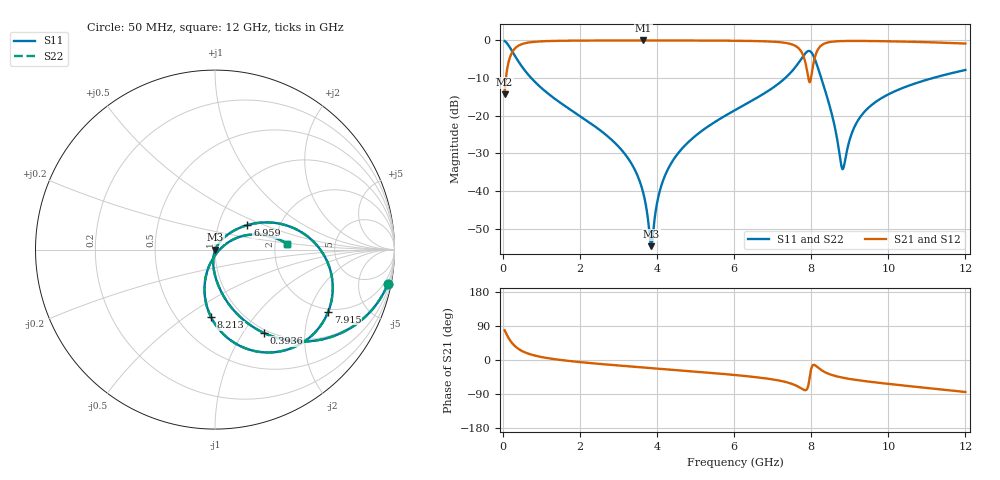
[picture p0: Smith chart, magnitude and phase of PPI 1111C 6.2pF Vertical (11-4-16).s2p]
# GHz S MA R 50
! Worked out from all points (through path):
!   1601 points, 50 MHz to 12 GHz, reference 50 ohm
!   highest |S21| = -0.02 dB at 3.65 GHz (marker M1); lowest = -14.3 dB at 50 MHz (marker M2)
!   group delay of S21, straight-line fit = 22.8 ps
!   lowest |S11| = -54.6 dB at 3.852 GHz (marker M3), VSWR 1.00, Z = 50.2 - j0.0771 ohm
!   |S11| at or under -10 dB: 741.6 MHz to 7.326 GHz (6.585 GHz wide, 163 % of centre); 8.262 GHz to 11.15 GHz (2.891 GHz wide, 29.8 % of centre)
!   |S22| runs from -54.6 to -0.2 dB; largest |S21 - S12| = 0
!   S11 on the Smith chart (normalised r, x): 50 MHz: 0.95, -9.92; 393.6 MHz: 0.95, -1.25; 6.959 GHz: 1.37, +0.40; 7.915 GHz: 1.89, -2.70; 8.213 GHz: 0.72, -0.64; 12 GHz: 2.34, +0.18
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0.05  0.9812 -11.4  0.1929 78.6  0.1929 78.6  0.9812 -11.4
0.1919063  0.7976 -38.2  0.6029 51.8  0.6029 51.8  0.7976 -38.2
0.3935625  0.5396 -59.5  0.8414 30.4  0.8414 30.4  0.5396 -59.5
0.8715625  0.2701 -79.0  0.9619 10.8  0.9619 10.8  0.2701 -79.0
2.044156  0.09594 -95.2  0.994 -5.9  0.994 -5.9  0.09594 -95.2
3.142063  0.03237 -102.8  0.9977 -15.6  0.9977 -15.6  0.03237 -102.8
3.649938  0.009261 -98.6  0.998 -19.7  0.998 -19.7  0.009261 -98.6
3.851594  0.001859 -24.4  0.9979 -21.3  0.9979 -21.3  0.001859 -24.4
4.038312  0.008458 54.0  0.9978 -22.8  0.9978 -22.8  0.008458 54.0
4.269844  0.01881 59.2  0.9975 -24.7  0.9975 -24.7  0.01881 59.2
4.643281  0.03626 58.9  0.9969 -27.7  0.9969 -27.7  0.03626 58.9
6.025  0.1187 48.6  0.9889 -39.6  0.9889 -39.6  0.1187 48.6
6.958594  0.2261 37.1  0.9646 -50.6  0.9646 -50.6  0.2261 37.1
7.63825  0.4757 13.1  0.8157 -69.0  0.8157 -69.0  0.4757 13.1
7.914594  0.7194 -28.7  0.3437 -71.4  0.3437 -71.4  0.7194 -28.7
8.019156  0.679 -56.2  0.3743 -17.7  0.3743 -17.7  0.679 -56.2
8.213344  0.3778 -93.3  0.8079 -22.8  0.8079 -22.8  0.3778 -93.3
8.5345  0.1058 -109.9  0.9592 -39.4  0.9592 -39.4  0.1058 -109.9
8.818312  0.01953 -38.8  0.9802 -46.7  0.9802 -46.7  0.01953 -38.8
9.236562  0.0904 29.0  0.9838 -53.6  0.9838 -53.6  0.0904 29.0
10.01331  0.1935 24.6  0.9728 -63.1  0.9728 -63.1  0.1935 24.6
12  0.4047 4.6  0.9073 -84.5  0.9073 -84.5  0.4047 4.6
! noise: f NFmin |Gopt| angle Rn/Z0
0.05  0.0004172  0.8906  2.449  0.0008296
1.372  0.003764  0.6753  8.451  0.002224
2.701  0.006217  0.6278  15.42  0.003077
4.031  0.008613  0.6104  22.26  0.003956
5.36  0.01164  0.6231  28.87  0.005434
6.682  0.01936  0.711  35.49  0.01201
8.012  0.3248  0.9769  42.68  2.782
9.341  0.02879  0.7425  48.65  0.01871
10.67  0.02457  0.6818  53.72  0.01201
12  0.02565  0.6749  58.55  0.01171
